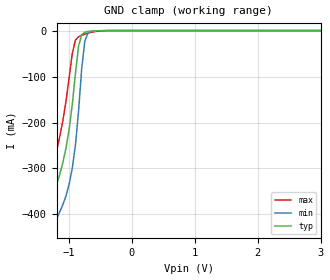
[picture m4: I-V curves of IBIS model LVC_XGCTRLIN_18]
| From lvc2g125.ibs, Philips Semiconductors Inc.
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|   Model LVC_XGCTRLIN_18
[Model]   LVC_XGCTRLIN_18
Model_type   Input
Vinl =   0.63V
Vinh =   1.17V
C_comp   3.07pF   2.35pF   3.88pF
[Model Spec]
| Note: The input and output voltage ratings may be exceeded if the input and
|   output current ratings are observed (please refer to the data sheet)
|   Subparameter   typ   min   max
| Thresholds
Vinh   1.17   1.0725   1.2675
Vinl   0.63   0.5775   0.6825
| Overshoot
S_overshoot_high   6.5   6.5   6.5   | Static overshoot
S_overshoot_low   -0.5   -0.5   -0.5
D_overshoot_high   7.2   7.2   7.2   | Dynamic overshoot
D_overshoot_low   -0.95   -0.9   -1.0
D_overshoot_time   3n   3n   3n
|Ambient temperature:   25   85   -40
[Temperature Range]   25   85   -40
[Voltage Range]   1.80V   1.65V   1.95V
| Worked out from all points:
|   GND clamp passes 1 mA (typ) near -0.62 V on its own axis
|Process Range   nominal   slow   fast
[GND_clamp]
| voltage   I(typ)   I(min)   I(max)
-5.5V     -4.545A    -4.602A    -4.489A
-1.45V    -537.1mA   -602.6mA   -471.2mA
-1.4V     -490mA     -555.7mA   -423.8mA
-1.35V    -443.6mA   -509.7mA   -377.2mA
-1.25V    -361.5mA   -430.2mA   -292.5mA
-1.1V     -287.7mA   -378.9mA   -196.8mA
-1V       -214.9mA   -334.5mA   -102.9mA
-950mV    -161.3mA   -299.8mA   -50.33mA
-850mV    -34.09mA   -175.9mA   -13.26mA
-750mV    -3.481mA   -22.77mA   -7.786mA
-550mV    -515.4uA   -351.6uA   -1.398mA
5.5V      118.2pA    1.085nA    8.619pA
